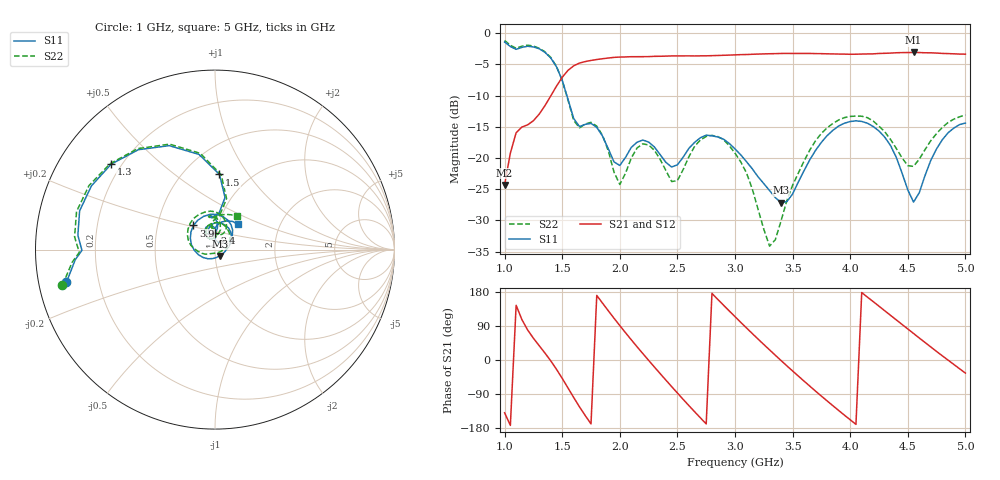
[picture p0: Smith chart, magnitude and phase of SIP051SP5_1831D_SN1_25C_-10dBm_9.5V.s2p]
# GHz  S  dB  R  50
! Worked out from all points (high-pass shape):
!   81 points, 1 GHz to 5 GHz, reference 50 ohm
!   highest |S21| = -3.11 dB at 4.55 GHz (marker M1); lowest = -24.3 dB at 1 GHz (marker M2)
!   |S21| within 3 dB of the highest: 1.544 GHz to end of sweep
!   lowest |S11| = -27.2 dB at 3.4 GHz (marker M3), VSWR 1.09, Z = 52.6 - j3.67 ohm
!   |S11| at or under -10 dB: 1.54 GHz to end of sweep
!   |S22| runs from -34.1 to -1.2 dB; largest |S21 - S12| = 0.0023
!   S11 on the Smith chart (normalised r, x): 1 GHz: 0.08, -0.11; 1.3 GHz: 0.16, +0.35; 1.5 GHz: 0.73, +0.74; 2.4 GHz: 0.98, +0.18; 3.9 GHz: 0.76, +0.21; 5 GHz: 1.23, +0.36
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1  -1.43 -167.5  -24.31 -139.3  -24.33 -139.6  -1.18 -166.9
1.1  -2.60 -179.7  -15.96 144.3  -15.97 144.2  -2.42 -178.8
1.3  -2.51 140.5  -12.98 37.9  -12.97 37.9  -2.43 140.8
1.5  -7.55 86.6  -7.08 -48.3  -7.08 -48.4  -7.58 85.2
1.7  -14.61 100.4  -4.56 -146.8  -4.56 -146.6  -14.56 101.4
1.85  -16.50 84.9  -4.11 150.0  -4.10 149.9  -16.38 79.1
2  -21.20 108.0  -3.84 90.8  -3.83 90.8  -24.24 104.5
2.2  -17.13 104.7  -3.78 16.9  -3.78 16.9  -17.74 109.1
2.35  -19.46 88.2  -3.71 -35.8  -3.71 -35.8  -20.23 86.5
2.4  -20.70 89.7  -3.69 -53.0  -3.69 -53.1  -22.00 87.9
2.55  -19.87 110.2  -3.65 -103.9  -3.65 -103.8  -21.85 120.8
2.75  -16.35 85.1  -3.64 -168.6  -3.63 -168.6  -16.55 95.8
3  -18.55 39.1  -3.49 114.4  -3.48 114.4  -19.23 39.8
3.3  -25.22 -14.5  -3.31 26.7  -3.31 26.7  -34.12 -69.8
3.4  -27.15 -52.5  -3.26 -1.4  -3.26 -1.4  -30.06 -134.9
3.7  -18.76 -178.1  -3.29 -82.3  -3.28 -82.2  -17.21 169.5
3.9  -14.88 131.7  -3.36 -133.2  -3.36 -133.3  -13.91 133.5
4.1  -14.15 87.2  -3.36 178.0  -3.35 178.0  -13.31 96.7
4.35  -18.00 40.0  -3.21 117.9  -3.20 117.9  -17.02 62.6
4.55  -27.06 61.6  -3.11 70.0  -3.11 69.9  -21.34 81.5
4.8  -17.07 84.2  -3.26 10.9  -3.25 11.0  -15.10 88.4
5  -14.41 48.7  -3.38 -34.5  -3.38 -34.5  -13.12 56.7
